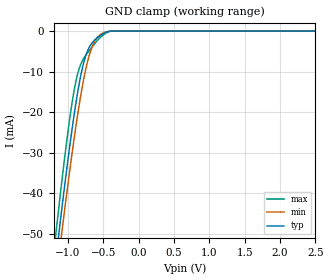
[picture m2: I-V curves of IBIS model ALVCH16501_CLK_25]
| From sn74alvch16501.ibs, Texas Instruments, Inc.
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[Model]   ALVCH16501_CLK_25
Model_type  Input
Vinl=0.7
Vinh=1.7
| variable   typ   min   max
C_comp   1.11pF   0.82pF   1.23pF
[Temperature Range]   40   100   -40
| Ambient temperature   25   85   -40
[Voltage range]   2.5   2.3   2.7
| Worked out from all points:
|   GND clamp passes 1 mA (typ) near -0.53 V on its own axis
[GND Clamp]
| ALVCH16501_CLK_25
|   Voltage   I(typ)   I(min)   I(max)
-2.5V     -275.2mA   -274.4mA   -278.8mA
-1.165V   -55.41mA   -61.03mA   -49.06mA
-1.13V    -50.2mA    -55.94mA   -43.64mA
-1.085V   -43.62mA   -49.51mA   -36.85mA
-925mV    -22.12mA   -28.06mA   -15.89mA
-865mV    -15.36mA   -20.9mA    -10.69mA
-800mV    -9.434mA   -14.01mA   -7.465mA
-740mV    -5.665mA   -8.789mA   -5.778mA
-665mV    -3.059mA   -4.2mA     -4.065mA
-520mV    -856uA     -629.9uA   -1.227mA
-375mV    -1.864uA   -31.43uA   -304.7nA
2.5V      913.9pA    48.35nA    15.21pA
